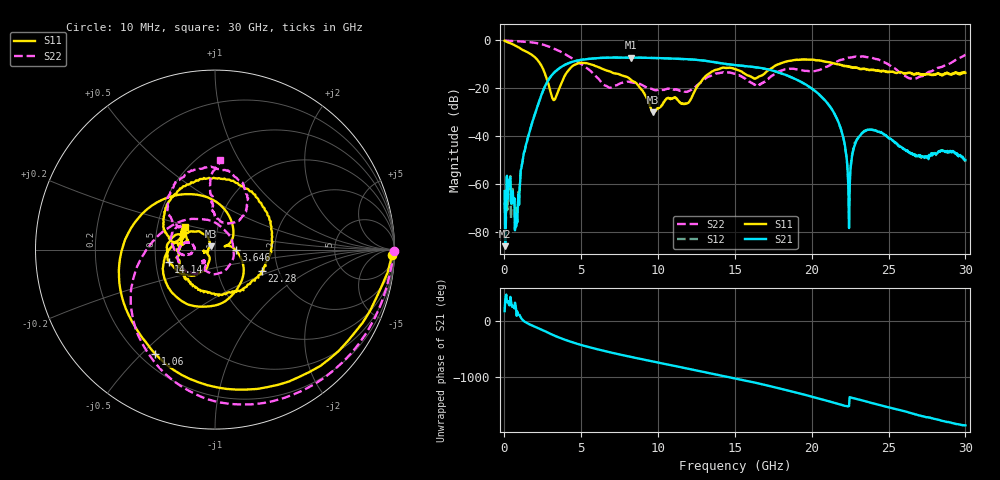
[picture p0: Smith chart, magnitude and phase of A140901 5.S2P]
!  2-Port S-parameters saved by WinCal
! VAR MeasName=S-Parameters (CALIBRATED_DATA) read from VNA (N5244A)
! VAR MeasDate=11/3/2014 9:26:55 AM
! VAR NAME=A140901 5
! VAR FILENAME=A140901 5.S2P
! VAR DATE=11/3/2014 9:26:55 AM
! VAR PHYS_PORTS=1,2
# Hz S RI R 50
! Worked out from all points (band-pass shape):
!   801 points, 10 MHz to 30 GHz, reference 50 ohm
!   highest |S21| = -7.14 dB at 8.257 GHz (marker M1); lowest = -86.0 dB at 47.49 MHz (marker M2)
!   |S21| within 3 dB of the highest: 3.958 GHz to 14.79 GHz (10.83 GHz wide, 116 % of centre)
!   lowest |S11| = -30.1 dB at 9.682 GHz (marker M3), VSWR 1.06, Z = 47.5 + j1.8 ohm
!   |S11| at or under -10 dB: 2.353 GHz to 4.633 GHz (2.28 GHz wide, 65.3 % of centre); 5.647 GHz to 17.82 GHz (12.17 GHz wide, 104 % of centre); 21.72 GHz to end of sweep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
!   |S22| runs from -21.5 to 0.0 dB; largest |S21 - S12| = 0.0038
!   S11 on the Smith chart (normalised r, x): 10 MHz: 22, -54; 1.06 GHz: 0.26, -0.55; 3.646 GHz: 1.26, -0.01; 14.14 GHz: 0.59, -0.09; 22.28 GHz: 1.63, -0.43; 30 GHz: 0.69, +0.19
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1e7  0.9866 -0.0312  -0.00071 1.93e-05  -0.000134 0.000386  0.9982 -0.00789
4.74875e7  0.9617 -0.1277  5e-05 -2.76e-06  -0.000185 0.000144  0.9936 -0.0371
7.972375e8  -0.0411 -0.7557  -2.5e-05 0.000229  -0.000164 0.00024  0.8375 -0.473
1.05965e9  -0.332 -0.5828  0.000568 0.00188  0.00051 0.0018  0.7396 -0.5981
2.184275e9  -0.2315 0.2997  -0.0241 -0.0383  -0.024 -0.0381  0.1066 -0.8612
3.15895e9  0.0561 0.0181  -0.076 0.1859  -0.0759 0.1852  -0.3743 -0.5756
3.646288e9  0.1148 -0.00208  0.1479 0.2287  0.1476 0.2284  -0.4634 -0.3539
5.033325e9  -0.1848 -0.2872  0.1384 -0.3688  0.1383 -0.3693  -0.3011 0.0909
6.6078e9  -0.2354 0.025  -0.4351 0.00463  -0.4343 0.00471  0.0845 0.0745
8.25725e9  -0.1079 0.1007  0.0876 0.4306  0.0874 0.4287  -0.0295 -0.129
9.681775e9  -0.025 0.0189  0.4289 -0.0265  0.4282 -0.0256  -0.0616 -0.0701
1.001916e10  -0.0389 -0.0051  0.3953 -0.1642  0.3942 -0.1638  -0.0622 -0.0708
1.241836e10  -0.0396 -0.0839  -0.368 -0.1439  -0.3686 -0.1431  -0.0527 -0.0929
1.414279e10  -0.2578 -0.0678  -0.0765 0.3234  -0.0769 0.3244  -0.1954 -0.0874
1.5005e10  -0.2452 0.0577  0.1721 0.2524  0.173 0.25  -0.1998 0.00677
1.714179e10  -0.2304 0.0421  0.0668 -0.2389  0.0667 -0.2378  -0.1516 -0.0288
2.002832e10  0.0797 0.3898  0.00548 0.0971  0.00497 0.097  -0.1841 0.1243
2.167778e10  0.3146 0.03  0.0168 -0.0137  0.017 -0.0135  -0.2632 0.2538
2.227758e10  0.2593 -0.1206  0.000525 -0.00329  0.000451 -0.00333  -0.2293 0.3615
2.336471e10  0.039 -0.253  0.0117 0.00318  0.012 0.00319  -0.0212 0.4627
2.501416e10  -0.1837 -0.1133  -0.00216 -0.00873  -0.00227 -0.00889  0.1816 0.2558
3e10  -0.1664 0.1274  0.0013 -0.00288  0.00116 -0.00265  0.03 0.4976
